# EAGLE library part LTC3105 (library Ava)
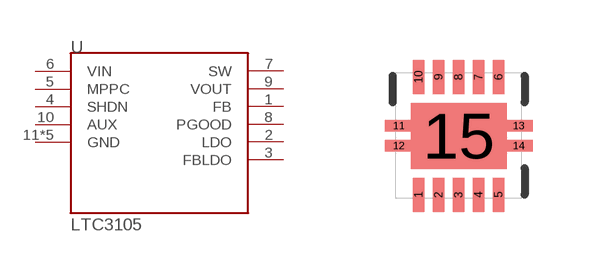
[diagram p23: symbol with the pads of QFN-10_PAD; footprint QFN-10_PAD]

Designator prefix -

## LTC3105  [QFN-10_PAD]
1  FB  pas
2  LDO  sup
3  FBLDO  sup
4  SHDN  in
5  MPPC  in
6  VIN  sup
7  SW  pas
8  PGOOD  pas
9  VOUT  pas
10  AUX  pas
11  GND  sup
12  GND  sup
13  GND  sup
14  GND  sup
15  GND  sup

## Footprint QFN-10_PAD (pad centres in mm)
smd 0.297 x 0.85: 1 -1,-1.475; 2 -0.5,-1.475; 3 0,-1.475; 4 0.5,-1.475; 5 1,-1.475; 6 1,1.475; 7 0.5,1.475; 8 0,1.475; 9 -0.5,1.475; 10 -1,1.475
smd 0.7 x 0.28: 11 -1.5,0.25; 12 -1.5,-0.25; 13 1.5,0.25; 14 1.5,-0.25
smd 2.4 x 1.65: 15 0,0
